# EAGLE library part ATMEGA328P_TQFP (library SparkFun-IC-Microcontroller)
Popular 328P in QFP Storefront component: ATmega328 - TQFP (COM-13448) Datasheet SparkFun Products SparkFun RedBoard - Programmed with Arduino (DEV-12757) Arduino Pro Mini 328 - 5V/16MHz (DEV-11113) Arduino Pro Mini 328 - 3.3V/8MHz (DEV-11114) SparkFun OpenLog (DEV-13712) SparkFun MicroView - OLED Arduino Module (DEV-12923) SparkFun Digital Sandbox (DEV-12651) SparkFun PicoBoard (WIG-11888) Arduino Fio (DEV-10116) LilyPad Arduino 328 Main Board (DEV-13342) SparkFun RedStick (DEV-13741) LilyPad MP3 (DEV-11013) LilyPad Arduino SimpleSnap (DEV-10941) SparkFun Stepoko (ROB-13899) SparkFun Geiger Counter (SEN-11345) SparkFun EL Sequencer (COM-12781) Arduino Pro 328 - 5V/16MHz (DEV-10915) CryptoCape (DEV-12773) SparkFun IR Thermometer Evaluation Board - MLX90614 (SEN-10740) SparkFun RedBot Mainboard (ROB-12097) Arduino Pro 328 - 3.3V/8MHz (DEV-10914) SparkFun Block for Intel® Edison - Arduino (DEV-13036) SparkFun Simon Says - Surface Mount Soldering Kit (KIT-10935) SparkFun 7-Segment Serial Display - Red (COM-11441) SparkFun 7-Segment Serial Display - White (COM-11629) SparkFun 7-Segment Serial Display - Yellow (COM-11443) SparkFun 7-Segment Serial Display - Kelly Green (COM-11440) SparkFun 7-Segment Serial Display - Blue (COM-11442) SparkFun OpenSegment Serial Display - 20mm (Blue) (COM-11647) SparkFun OpenSegment Serial Display - 20mm (Green) (COM-11646) SparkFun OpenSegment Serial Display - 20mm (White) (COM-11648) SparkFun OpenSegment Serial Display - 20mm (Red) (COM-11644)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
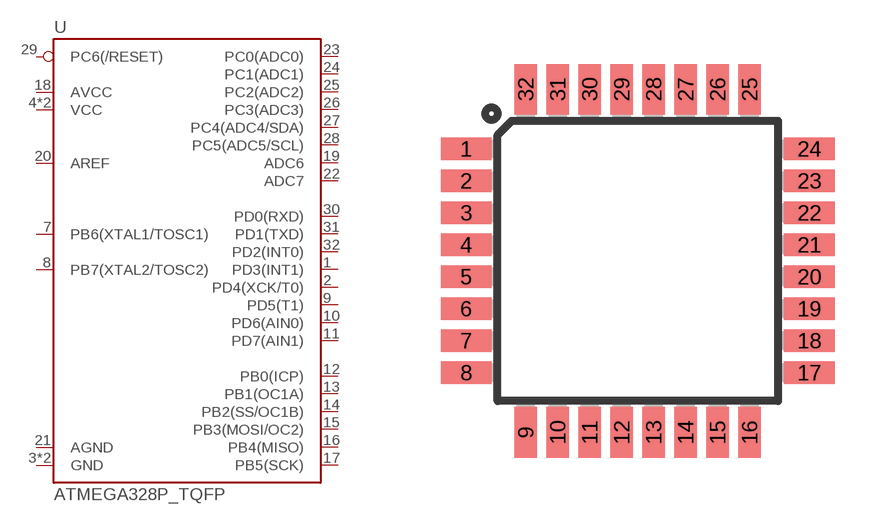
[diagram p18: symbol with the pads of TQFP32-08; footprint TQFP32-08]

Designator prefix U

## ATMEGA328P_TQFP (PROD_ID: IC-09069; VALUE: ATMEGA328P_TQFP)  [TQFP32-08]
1  PD3(INT1)
2  PD4(XCK/T0)
3  GND
4  VCC
5  GND
6  VCC
7  PB6(XTAL1/TOSC1)
8  PB7(XTAL2/TOSC2)
9  PD5(T1)
10  PD6(AIN0)
11  PD7(AIN1)
12  PB0(ICP)
13  PB1(OC1A)
14  PB2(SS/OC1B)
15  PB3(MOSI/OC2)
16  PB4(MISO)
17  PB5(SCK)
18  AVCC
19  ADC6
20  AREF
21  AGND
22  ADC7
23  PC0(ADC0)
24  PC1(ADC1)
25  PC2(ADC2)
26  PC3(ADC3)
27  PC4(ADC4/SDA)
28  PC5(ADC5/SCL)
29  PC6(/RESET)
30  PD0(RXD)
31  PD1(TXD)
32  PD2(INT0)

## Footprint TQFP32-08 (pad centres in mm)
Thin Plasic Quad Flat Package Grid 0.8 mm
smd 1.27 x 0.559: 1 -4.293,2.8; 2 -4.293,2; 3 -4.293,1.2; 4 -4.293,0.4; 5 -4.293,-0.4; 6 -4.293,-1.2; 7 -4.293,-2; 8 -4.293,-2.8; 17 4.293,-2.8; 18 4.293,-2; 19 4.293,-1.2; 20 4.293,-0.4; 21 4.293,0.4; 22 4.293,1.2; 23 4.293,2; 24 4.293,2.8
smd 0.559 x 1.27: 9 -2.8,-4.293; 10 -2,-4.293; 11 -1.2,-4.293; 12 -0.4,-4.293; 13 0.4,-4.293; 14 1.2,-4.293; 15 2,-4.293; 16 2.8,-4.293; 25 2.8,4.293; 26 2,4.293; 27 1.2,4.293; 28 0.4,4.293; 29 -0.4,4.293; 30 -1.2,4.293; 31 -2,4.293; 32 -2.8,4.293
